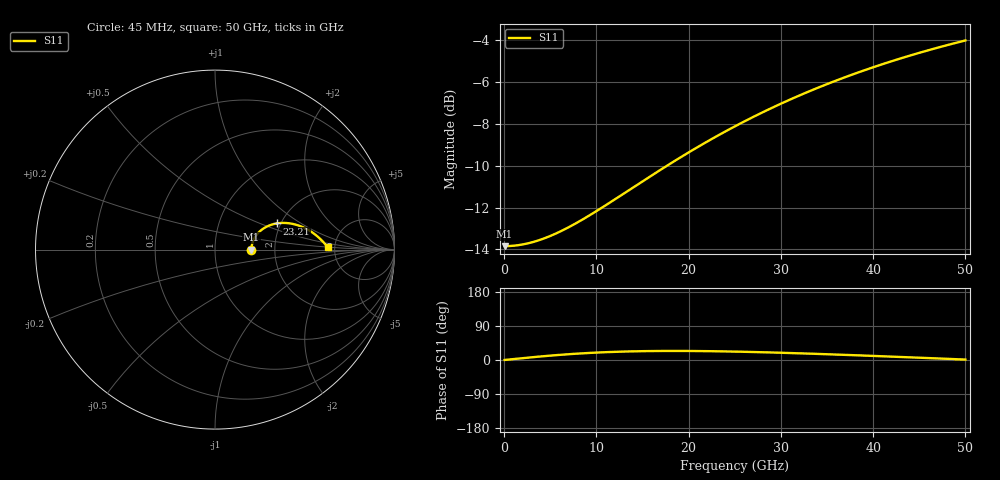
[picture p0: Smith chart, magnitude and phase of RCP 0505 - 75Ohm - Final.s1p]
!Vishay Electro-Films Inc.
!RCP Family
!Case Size 0505
!Assembly Style Surface Mount
!11/2/2015
!efi@vishay.com
# GHz S MA R 50
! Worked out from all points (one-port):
!   801 points, 45 MHz to 50 GHz, reference 50 ohm
!   lowest |S11| = -13.8 dB at 45 MHz (marker M1), VSWR 1.51, Z = 75.5 + j0.062 ohm
!   |S11| at or under -10 dB: start of sweep to 17.68 GHz
!   S11 on the Smith chart (normalised r, x): 45 MHz: 1.51, +0.00; 23.21 GHz: 1.90, +0.64; 50 GHz: 4.37, +0.18
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0.045  0.2032 0.1
1.54365  0.2043 3.8
3.0423  0.2076 7.3
4.603394  0.2131 10.8
6.289375  0.2214 14.1
7.53825  0.2288 16.2
8.912012  0.2381 18.2
10.72288  0.252 20.4
12.53375  0.2673 22.0
15.71838  0.2969 23.6
18.77812  0.3274 24.0
21.0261  0.3505 23.7
23.21163  0.3733 23.0
25.0225  0.3923 22.2
26.58359  0.4086 21.3
28.14469  0.4249 20.4
29.70578  0.441 19.4
31.26687  0.457 18.2
32.82797  0.4728 17.0
34.38906  0.4884 15.8
35.95016  0.5038 14.4
37.51125  0.5188 13.1
40.57099  0.5476 10.3
43.75563  0.5762 7.3
45.50405  0.5913 5.6
47.25247  0.606 3.9
49.25068  0.6223 1.9
50  0.6282 1.1
